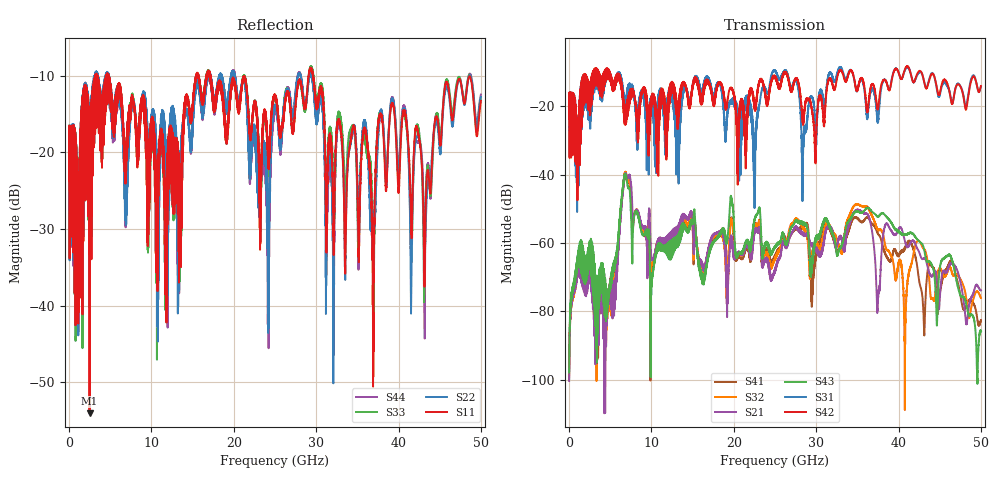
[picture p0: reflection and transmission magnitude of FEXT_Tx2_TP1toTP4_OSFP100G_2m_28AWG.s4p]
! Touchstone data
! Created: 27-Feb-2019 by IdEM 12 (12.1.0)
! COMMENTS
!  Created Wed Feb 27 12:03:36 2019
!  64 Port Network Data from SP1.SP block
!  freq  magS1_1  angS1_1  magS1_2  angS1_2  magS1_3  angS1_3  magS1_4  angS1_4
!  magS1_5  angS1_5  magS1_6  angS1_6  magS1_7  angS1_7  magS1_8  angS1_8
!  magS1_9  angS1_9  magS1_10  angS1_10  magS1_11  angS1_11  magS1_12  angS1_12
!  magS1_13  angS1_13  magS1_14  angS1_14  magS1_15  angS1_15  magS1_16  angS1_16
!  magS1_17  angS1_17  magS1_18  angS1_18  magS1_19  angS1_19  magS1_20  angS1_20
!  magS1_21  angS1_21  magS1_22  angS1_22  magS1_23  angS1_23  magS1_24  angS1_24
!  magS1_25  angS1_25  magS1_26  angS1_26  magS1_27  angS1_27  magS1_28  angS1_28
!  magS1_29  angS1_29  magS1_30  angS1_30  magS1_31  angS1_31  magS1_32  angS1_32
!  magS1_33  angS1_33  magS1_34  angS1_34  magS1_35  angS1_35  magS1_36  angS1_36
!  magS1_37  angS1_37  magS1_38  angS1_38  magS1_39  angS1_39  magS1_40  angS1_40
!  magS1_41  angS1_41  magS1_42  angS1_42  magS1_43  angS1_43  magS1_44  angS1_44
!  magS1_45  angS1_45  magS1_46  angS1_46  magS1_47  angS1_47  magS1_48  angS1_48
!  magS1_49  angS1_49  magS1_50  angS1_50  magS1_51  angS1_51  magS1_52  angS1_52
!  magS1_53  angS1_53  magS1_54  angS1_54  magS1_55  angS1_55  magS1_56  angS1_56
!  magS1_57  angS1_57  magS1_58  angS1_58  magS1_59  angS1_59  magS1_60  angS1_60
!  magS1_61  angS1_61  magS1_62  angS1_62  magS1_63  angS1_63  magS1_64  angS1_64
!  magS2_1  angS2_1  magS2_2  angS2_2  magS2_3  angS2_3  magS2_4  angS2_4
!  magS2_5  angS2_5  magS2_6  angS2_6  magS2_7  angS2_7  magS2_8  angS2_8
!  magS2_9  angS2_9  magS2_10  angS2_10  magS2_11  angS2_11  magS2_12  angS2_12
!  magS2_13  angS2_13  magS2_14  angS2_14  magS2_15  angS2_15  magS2_16  angS2_16
!  magS2_17  angS2_17  magS2_18  angS2_18  magS2_19  angS2_19  magS2_20  angS2_20
!  magS2_21  angS2_21  magS2_22  angS2_22  magS2_23  angS2_23  magS2_24  angS2_24
!  magS2_25  angS2_25  magS2_26  angS2_26  magS2_27  angS2_27  magS2_28  angS2_28
!  magS2_29  angS2_29  magS2_30  angS2_30  magS2_31  angS2_31  magS2_32  angS2_32
!  magS2_33  angS2_33  magS2_34  angS2_34  magS2_35  angS2_35  magS2_36  angS2_36
!  magS2_37  angS2_37  magS2_38  angS2_38  magS2_39  angS2_39  magS2_40  angS2_40
!  magS2_41  angS2_41  magS2_42  angS2_42  magS2_43  angS2_43  magS2_44  angS2_44
!  magS2_45  angS2_45  magS2_46  angS2_46  magS2_47  angS2_47  magS2_48  angS2_48
!  magS2_49  angS2_49  magS2_50  angS2_50  magS2_51  angS2_51  magS2_52  angS2_52
!  magS2_53  angS2_53  magS2_54  angS2_54  magS2_55  angS2_55  magS2_56  angS2_56
!  magS2_57  angS2_57  magS2_58  angS2_58  magS2_59  angS2_59  magS2_60  angS2_60
!  magS2_61  angS2_61  magS2_62  angS2_62  magS2_63  angS2_63  magS2_64  angS2_64
!  magS3_1  angS3_1  magS3_2  angS3_2  magS3_3  angS3_3  magS3_4  angS3_4
!  magS3_5  angS3_5  magS3_6  angS3_6  magS3_7  angS3_7  magS3_8  angS3_8
!  magS3_9  angS3_9  magS3_10  angS3_10  magS3_11  angS3_11  magS3_12  angS3_12
!  magS3_13  angS3_13  magS3_14  angS3_14  magS3_15  angS3_15  magS3_16  angS3_16
!  magS3_17  angS3_17  magS3_18  angS3_18  magS3_19  angS3_19  magS3_20  angS3_20
!  magS3_21  angS3_21  magS3_22  angS3_22  magS3_23  angS3_23  magS3_24  angS3_24
!  magS3_25  angS3_25  magS3_26  angS3_26  magS3_27  angS3_27  magS3_28  angS3_28
!  magS3_29  angS3_29  magS3_30  angS3_30  magS3_31  angS3_31  magS3_32  angS3_32
!  magS3_33  angS3_33  magS3_34  angS3_34  magS3_35  angS3_35  magS3_36  angS3_36
!  magS3_37  angS3_37  magS3_38  angS3_38  magS3_39  angS3_39  magS3_40  angS3_40
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# Hz S MA R 50
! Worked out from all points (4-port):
!   5000 points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, 10 MHz to 50 GHz, reference 50 ohm
!   strongest paths, dB at 10 MHz, 12.51 GHz, 25.01 GHz, 37.51 GHz, 50 GHz:
!     S42: -18.0, -13.8, -11.3, -20.6, -14.1
!     S31: -18.0, -16.4, -9.6, -24.1, -14.3
!     S43: -97.9, -62.2, -61.1, -52.3, -85.9
!     S21: -100.4, -59.0, -67.6, -76.4, -73.9
!     S32: -98.7, -60.5, -64.5, -56.3, -76.1
!     S41: -99.8, -60.3, -63.7, -57.4, -82.6
!   lowest |S11| = -54.1 dB at 2.49 GHz (marker M1), VSWR 1.00, Z = 49.8 + j0.0446 ohm
!   |S11| at or under -10 dB: 4.81 GHz to 15.41 GHz (10.6 GHz wide, 105 % of centre); 17.19 GHz to 29.09 GHz (11.9 GHz wide, 51.4 % of centre); 29.64 GHz to end of sweep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
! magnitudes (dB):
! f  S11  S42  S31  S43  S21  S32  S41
! 10 MHz  -17.7  -18.0  -18.0  -97.9  -100.4  -98.7  -99.8
! 2.49 GHz  -54.1  -21.4  -22.3  -65.3  -67.6  -65.9  -67.3
! 4.93 GHz  -11.6  -10.5  -10.8  -72.3  -74.3  -74.9  -72.0
! 7.06 GHz  -18.2  -20.8  -16.7  -42.7  -41.1  -41.7  -41.9
! 10.06 GHz  -15.5  -16.9  -17.3  -71.3  -65.0  -67.0  -67.4
! 36.28 GHz  -19.8  -21.1  -22.5  -49.8  -51.8  -49.7  -52.6
! 50 GHz  -13.3  -14.1  -14.3  -85.9  -73.9  -76.1  -82.6
